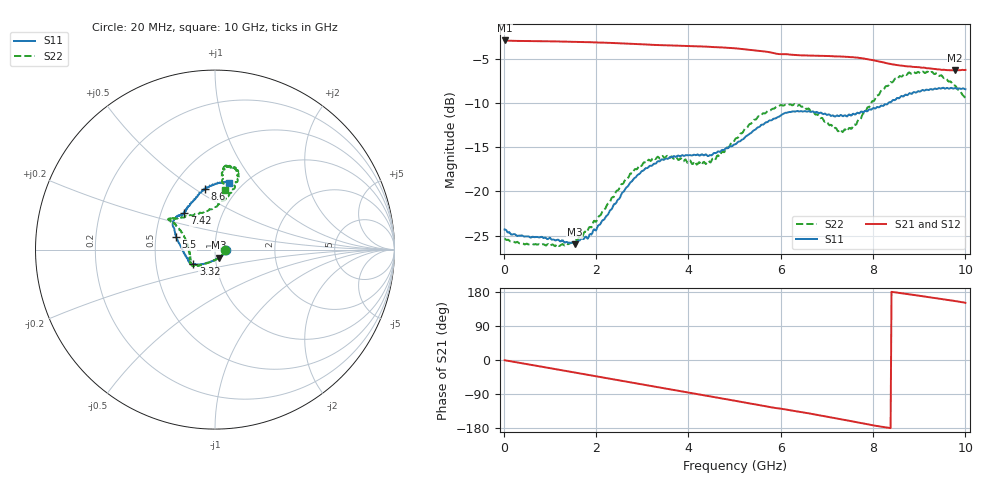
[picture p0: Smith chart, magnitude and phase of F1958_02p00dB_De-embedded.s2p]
! Integrated Device Technology
! Corporate Headquarters
! 6024 Silver Creek Valley Road
! San Jose, CA 95138  USA
! Phone:  1-408-284-8200
! Toll Free:  1-800-223-1366
! Webpage:  http://www.idt.com/
! Timing and RF Division
! 515 Groton Road, Suite 102
! Westford, MA 01886-6024
! Device:  F1958
! Description: 7-bit 0.25 dB Digital Step Attenuator
! Frequency:  0.001 -  6.000 GHz
! Package:  4x4 mm Thin QFN Plastic Package: 24 pin
! Ports:  2 RF, 12 DC
!  Pin  1  = D0
!  Pin  2  = VDD
!  Pin  3  = VMODE
!  Pin  4  = GND
!  Pin  5  = RF1  =  Port 1
!  Pin  6  = GND
!  Pin  7  = GND
!  Pin  8  = GND
!  Pin  9  = GND
!  Pin 10  = GND
!  Pin 11  = GND
!  Pin 12  = GND
!  Pin 13  = GND
!  Pin 14  = RF2  =  Port 2
!  Pin 15  = GND
!  Pin 16  = LE
!  Pin 17  = CLK
!  Pin 18  = DATA
!  Pin 19  = D6
!  Pin 20  = D5
!  Pin 21  = D4
!  Pin 22  = D3
!  Pin 23  = D2
!  Pin 24  = D1
! State:  8
! Atten State:  2.00 dB
! Voltage:  +3.30 Volts
! Current:  0.258 mA
! Data:  The device was measured on a F1958 evaluation board which has
!  individual transmission lines to the RF pins.  Data was collected
!  using a calibrated network analyzer.  The evaluation board was
!  de-embedded using Automatic Fixture Removal (AFR).
!  The reference plane is the edge of the package pin.
! Misc:
!  Action Tracker AT0419
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# GHz S dB R 50
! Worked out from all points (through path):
!   500 points, 20 MHz to 10 GHz, reference 50 ohm
!   highest |S21| = -2.96 dB at 20 MHz (marker M1); lowest = -6.3 dB at 9.78 GHz (marker M2)
!   group delay of S21, straight-line fit = 58.8 ps
!   lowest |S11| = -26.0 dB at 1.54 GHz (marker M3), VSWR 1.11, Z = 52.1 - j4.69 ohm
!   |S11| at or under -10 dB: start of sweep to 8.336 GHz
!   |S22| runs from -26.2 to -6.5 dB; largest |S21 - S12| = 0.0019
!   S11 on the Smith chart (normalised r, x): 20 MHz: 1.13, -0.01; 3.32 GHz: 0.78, -0.13; 5.5 GHz: 0.64, +0.10; 7.42 GHz: 0.66, +0.29; 8.6 GHz: 0.71, +0.55; 10 GHz: 0.87, +0.75
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0.02  -24.32 -2.3  -2.96 -0.6  -2.96 -0.5  -25.32 -2.6
1.1  -25.50 -35.8  -3.06 -23.6  -3.06 -23.6  -26.17 -44.6
1.54  -25.98 -63.2  -3.12 -33.1  -3.11 -33.0  -25.54 -75.6
1.7  -25.32 -74.3  -3.14 -36.4  -3.13 -36.4  -25.13 -87.0
2.02  -24.16 -98.8  -3.18 -43.3  -3.18 -43.3  -23.27 -107.1
2.78  -18.86 -134.0  -3.34 -59.6  -3.32 -59.7  -18.01 -135.2
3.32  -16.71 -145.7  -3.47 -71.1  -3.47 -71.2  -16.17 -145.9
3.36  -16.61 -145.6  -3.48 -72.0  -3.48 -72.1  -16.19 -145.0
4.34  -15.94 -160.0  -3.65 -92.8  -3.66 -92.9  -16.67 -175.6
4.62  -15.59 -166.9  -3.72 -98.9  -3.73 -98.9  -16.00 169.6
5.02  -14.69 178.4  -3.85 -107.7  -3.86 -107.7  -14.06 155.0
5.5  -12.79 161.8  -4.11 -118.2  -4.12 -118.2  -11.62 147.3
6  -11.43 150.8  -4.50 -128.4  -4.51 -128.4  -10.25 146.6
6.68  -10.99 138.8  -4.67 -142.3  -4.69 -142.2  -10.96 141.4
7.2  -11.48 132.7  -4.76 -153.7  -4.77 -153.6  -12.86 119.0
7.42  -11.51 130.2  -4.81 -158.9  -4.82 -158.8  -13.15 103.4
7.94  -10.76 118.7  -5.13 -171.1  -5.13 -171.1  -10.31 76.0
8.34  -9.97 107.7  -5.57 -179.1  -5.57 -179.2  -7.99 71.7
8.6  -9.27 99.7  -5.79 176.4  -5.80 176.5  -7.01 74.2
9.26  -8.46 84.2  -6.14 164.7  -6.14 164.6  -6.54 81.7
9.78  -8.33 78.5  -6.34 155.5  -6.36 155.5  -8.06 83.7
10  -8.46 78.0  -6.28 150.8  -6.31 150.9  -9.48 80.3
